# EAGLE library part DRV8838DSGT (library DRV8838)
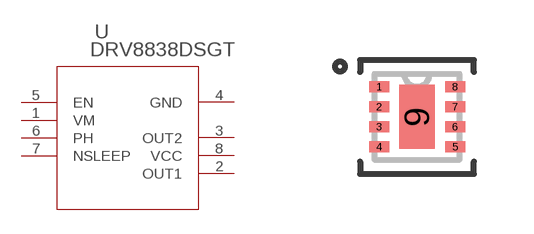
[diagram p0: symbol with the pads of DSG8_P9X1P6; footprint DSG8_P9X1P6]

Designator prefix U

## DRV8838DSGT (MANUFACTURER_PART_NUMBER: DRV8838DSGT; VENDOR: Texas Instruments)  [DSG8_P9X1P6]
1  VM  pwr
2  OUT1  out
3  OUT2  out
4  GND  pwr
5  EN  in
6  PH  in
7  NSLEEP  in
8  VCC  pwr

## Footprint DSG8_P9X1P6 (pad centres in mm)
smd 0.5 x 0.28: 1 -0.95,0.75; 2 -0.95,0.25; 3 -0.95,-0.25; 4 -0.95,-0.75; 5 0.95,-0.75; 6 0.95,-0.25; 7 0.95,0.25; 8 0.95,0.75
smd 0.889 x 1.6: 9 0,0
